|Texas Instruments Incorporated
|tmux8108, 100V 1 Channel 8:1 mux
[IBIS Ver]   4.1
[File name]   tmux8108.ibs
[Date]   08/12/21
[File Rev]   1.0
[Source]
| Texas Instruments Incorporated.
| ASC-INT-MPD
| 12500 TI Blvd
| Dallas, TX - 75243
[Notes]   Revision History:
| Rev 1.0: 08/12/21
| - Initial version of the model
| - Model generated from simulations in SPECTRE
| - C_comp although listed in numerical order of value are
|   obtained from varying PVT conditions. For PVT conditions for
|   each specific value refer the buffer description under
|   respective [Model]. IBIS model user is responsible for using
|   appropriate C_comp to simulate for Signal Integrity.
[Disclaimer]
| This model is designed as an aid for customers of Texas Instruments.
| TI and its licensors and suppliers make no warranties, either expressed
| or implied, with respect to this  model, including the warranties of
| merchantability or fitness for a particular purpose. The model is
| provided solely on an "as is" basis. The entire risk as to its quality
| and performance is with the customer.
| This model is subject to change without notice. Texas Instruments
| Incorporated is not responsible for updating this model.
[Copyright]
(C) Copyright 2021 Texas Instruments Incorporated.All rights reserved.
|  Component TMUX8108PW 16-pin - PW package
|  Part # TMUX8108PW
[Component]   TMUX8108PW
[Manufacturer]  TI
[Package]
|   typ   min   max
R_pkg   0.14389   NA   NA
L_pkg   1.96144nH   NA   NA
C_pkg   0.37623pF   NA   NA
[Pin]   signal_name   model_name
   1   A0   inbuf
   2   EN   inbuf
   3   VSS   power
   4   S1   sterm
   5   S2   sterm
   6   S3   sterm
   7   S4   sterm
   8   D   dterm
   9   S8   sterm
   10   S7   sterm
   11   S6   sterm
   12   S5   sterm
   13   VDD   power
   14   GND   gnd
   15   A2   inbuf
   16   A1   inbuf
[Series Switch Groups]
On 1 /
On 2 /
On 3 /
On 4 /
On 5 /
On 6 /
On 7 /
On 8 /
Off 1 2 3 4 5 6 7 8 /
[Series Pin Mapping]  pin_2 model_name function_table_group
|   4   8   switch_dual_50   1
|   5   8   switch_dual_50   2
|   6   8   switch_dual_50   3
|  7   8   switch_dual_50   4
|  12   8   switch_dual_50   5
|  11   8   switch_dual_50   6
|  10   8   switch_dual_50   7
|   9   8   switch_dual_50   8
|   4   8   switch_dual_15   1
|   5   8   switch_dual_15   2
|   6   8   switch_dual_15   3
|   7   8   switch_dual_15   4
|  12   8   switch_dual_15   5
|  11   8   switch_dual_15   6
|  10   8   switch_dual_15   7
|   9   8   switch_dual_15   8
|   4   8   switch_72   1
|   5   8   switch_72   2
|   6   8   switch_72   3
|   7   8   switch_72   4
|  12   8   switch_72   5
|  11   8   switch_72   6
|  10   8   switch_72   7
|   9   8   switch_72   8
|   4   8   switch_100   1
|   5   8   switch_100   2
|   6   8   switch_100   3
|   7   8   switch_100   4
|  12   8   switch_100   5
|  11   8   switch_100   6
|  10   8   switch_100   7
|   9   8   switch_100   8
   4   8   switch_dual_36   1
   5   8   switch_dual_36   2
   6   8   switch_dual_36   3
   7   8   switch_dual_36   4
  12   8   switch_dual_36   5
  11   8   switch_dual_36   6
  10   8   switch_dual_36   7
   9   8   switch_dual_36   8
|  Component TMUX8108RUM 16-pin - RUM package
|  Part # TMUX8108RUM
[Component]   TMUX8108RUM
[Manufacturer]  TI
[Package]
|   typ   min   max
R_pkg   0.1   NA   NA
L_pkg   1.0nH   NA   NA
C_pkg   0.2pF   NA   NA
[Pin]   signal_name   model_name
   1   VSS   power
   2   S1   sterm
   3   S2   sterm
   4   S3   sterm
   5   S4   sterm
   6   D   dterm
   7   S8   sterm
   8   S7   sterm
   9   S6   sterm
   10   S5   sterm
   11   VDD   power
   12   GND   gnd
   13   A2   inbuf
   14   A1   inbuf
   15   A0   inbuf
   16   EN   inbuf
[Series Switch Groups]
On 1 /
On 2 /
On 3 /
On 4 /
On 5 /
On 6 /
On 7 /
On 8 /
Off 1 2 3 4 5 6 7 8 /
[Series Pin Mapping]  pin_2 model_name function_table_group
|   2   6   switch_dual_50   1
|   3   6   switch_dual_50   2
|   4   6   switch_dual_50   3
|   5   6   switch_dual_50   4
|  10   6   switch_dual_50   5
|   9   6   switch_dual_50   6
|   8   6   switch_dual_50   7
|   7   6   switch_dual_50   8
|   2   6   switch_dual_15   1
|   3   6   switch_dual_15   2
|   4   6   switch_dual_15   3
|   5   6   switch_dual_15   4
|  10   6   switch_dual_15   5
|   9   6   switch_dual_15   6
|   8   6   switch_dual_15   7
|   7   6   switch_dual_15   8
|   2   6   switch_72   1
|   3   6   switch_72   2
|   4   6   switch_72   3
|   5   6   switch_72   4
|  10   6   switch_72   5
|   9   6   switch_72   6
|   8   6   switch_72   7
|   7   6   switch_72   8
|   2   6   switch_100   1
|   3   6   switch_100   2
|   4   6   switch_100   3
|   5   6   switch_100   4
|  10   6   switch_100   5
|   9   6   switch_100   6
|   8   6   switch_100   7
|   7   6   switch_100   8
   2   6   switch_dual_36   1
   3   6   switch_dual_36   2
   4   6   switch_dual_36   3
   5   6   switch_dual_36   4
  10   6   switch_dual_36   5
   9   6   switch_dual_36   6
   8   6   switch_dual_36   7
   7   6   switch_dual_36   8
[Model Selector] dterm
dterm_dual_50 Use for operation at +/-50V
dterm_dual_15 Use for operation at +/-15V
dterm_72 Use for operation at 72V
dterm_100 Use for operation at 100V
dterm_dual_36 Use for operation at +/-36V
[Model Selector] sterm
sterm_dual_50 Use for operation at +/-50V
sterm_dual_15 Use for operation at +/-15V
sterm_72 Use for operation at 72V
sterm_100 Use for operation at 100V
sterm_dual_36 Use for operation at +/-36V
[Model Selector] inbuf
inbuf_dual_50 Use for operation at +/-50V
inbuf_dual_15 Use for operation at +/-15V
inbuf_72 Use for operation at 72V
inbuf_100 Use for operation at 100V
inbuf_dual_36 Use for operation at +/-36V
| switch_dual_50
[Model]   switch_dual_50
Model_type   Series_switch
|   typ   min   max
C_comp   4.014581e-12   NA   NA
[Voltage Range]   50   NA   NA
[Power Clamp Reference]   50   NA   NA
[Temperature Range]   27   NA   NA
[On]
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[Off]
|   typ   min   max
[R Series]   10G   NA   NA
| switch_dual_15
[Model]   switch_dual_15
Model_type   Series_switch
|   typ   min   max
C_comp   4.014581e-12   NA   NA
[Voltage Range]   15   NA   NA
[Power Clamp Reference]   15   NA   NA
[Temperature Range]   27   NA   NA
[On]
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[Off]
|   typ   min   max
[R Series]   10G   NA   NA
| switch_72
[Model]   switch_72
Model_type   Series_switch
|   typ   min   max
C_comp   4.014581e-12   NA   NA
[Voltage Range]   72   NA   NA
[Power Clamp Reference]   72   NA   NA
[Temperature Range]   27   NA   NA
[On]
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[Off]
|   typ   min   max
[R Series]   10G   NA   NA
| switch_100
[Model]   switch_100
Model_type   Series_switch
|   typ   min   max
C_comp   4.014581e-12   NA   NA
[Voltage Range]   100   NA   NA
[Power Clamp Reference]   100   NA   NA
[Temperature Range]   27   NA   NA
[On]
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[Off]
|   typ   min   max
[R Series]   10G   NA   NA
| switch_dual_36
[Model]   switch_dual_36
Model_type   Series_switch
|   typ   min   max
C_comp   4.014581e-12   NA   NA
[Voltage Range]   36   NA   NA
[Power Clamp Reference]   36   NA   NA
[Temperature Range]   27   NA   NA
[On]
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[Off]
|   typ   min   max
[R Series]   10G   NA   NA
| Models and submodels in the file (20): dterm_dual_50 (Terminator), dterm_dual_15 (Terminator), dterm_72 (Terminator), dterm_100 (Terminator), dterm_dual_36 (Terminator), switch_dual_50 (Series_switch), switch_dual_15 (Series_switch), switch_72 (Series_switch), switch_100 (Series_switch), switch_dual_36 (Series_switch), sterm_dual_50 (Terminator), sterm_dual_15 (Terminator), sterm_72 (Terminator), sterm_100 (Terminator), sterm_dual_36 (Terminator), inbuf_dual_50 (Input), inbuf_dual_15 (Input), inbuf_72 (Input), inbuf_100 (Input), inbuf_dual_36 (Input)
